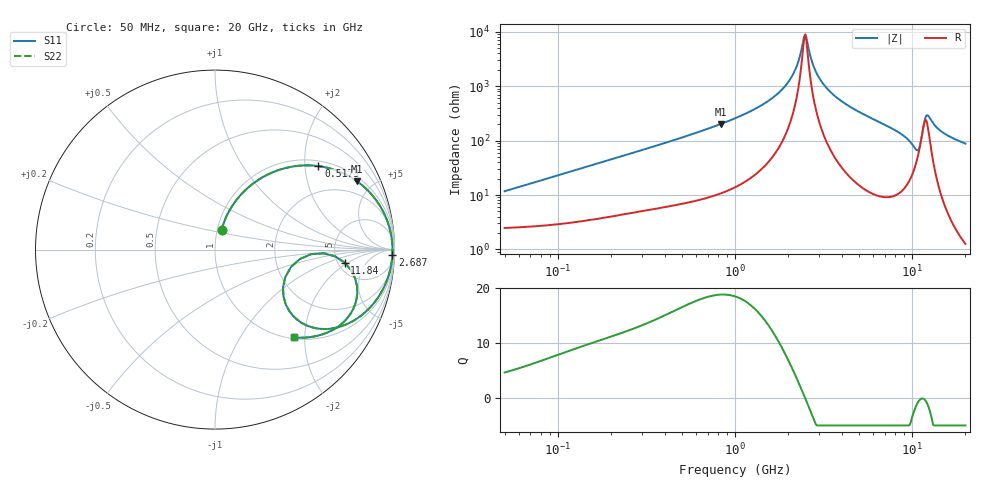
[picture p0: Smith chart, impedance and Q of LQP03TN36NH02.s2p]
!Murata Part Number: LQP03TN36NH02
!These Parameters are Measured in Series Mode Connection
!  o--[Z]--o
!Port1  Port2
!  o-------o
!Freq. Start=50[MHz] Stop=20[GHz], 401[Steps]
# Hz S RI R 50
!Freq.(Hz) S11(Real) S11(Imag) S21(Real) S21(Imag) S12(Real) S12(Imag) S22(Real) S22(Imag)
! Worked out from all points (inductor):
!   401 points, 50 MHz to 20 GHz, reference 50 ohm
!   read as one part in series: L = 36.4 nH near 51.52 MHz
!   highest Q = 18.8 at 835.5 MHz (marker M1), where L = 38.6 nH
!   self-resonance near 2.456 GHz
!   S11 on the Smith chart (normalised r, x): 50 MHz: 1.05, +0.23; 517.3 MHz: 1.14, +2.35; 2.687 GHz: 24, -60; 11.84 GHz: 5.75, -1.77; 20 GHz: 1.03, -1.76
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5e7  0.0363 0.1079  0.9637 -0.1079  0.9637 -0.1079  0.0363 0.1079
1.364002e8  0.1116 0.2661  0.8884 -0.2661  0.8884 -0.2661  0.1116 0.2661
3.721004e8  0.4169 0.4599  0.5831 -0.4599  0.5831 -0.4599  0.4169 0.4599
5.173368e8  0.5761 0.4652  0.4239 -0.4652  0.4239 -0.4652  0.5761 0.4652
8.354841e8  0.7926 0.3798  0.2074 -0.3798  0.2074 -0.3798  0.7926 0.3798
1e9  0.8552 0.3259  0.1448 -0.3259  0.1448 -0.3259  0.8552 0.3259
1.454215e9  0.9447 0.1964  0.0553 -0.1964  0.0553 -0.1964  0.9447 0.1964
1.875929e9  0.9767 0.1038  0.0233 -0.1038  0.0233 -0.1038  0.9767 0.1038
2.179053e9  0.9861 0.0489  0.0139 -0.0489  0.0139 -0.0489  0.9861 0.0489
2.493527e9  0.9889 -0.000672  0.0111 0.000672  0.0111 0.000672  0.9889 -0.000672
2.687447e9  0.9883 -0.0284  0.0117 0.0284  0.0117 0.0284  0.9883 -0.0284
2.728004e9  0.9879 -0.0339  0.0121 0.0339  0.0121 0.0339  0.9879 -0.0339
3.075291e9  0.9829 -0.0785  0.0171 0.0785  0.0171 0.0785  0.9829 -0.0785
3.736399e9  0.9649 -0.1522  0.0351 0.1522  0.0351 0.1522  0.9649 -0.1522
7.442007e9  0.7469 -0.4096  0.2531 0.4096  0.2531 0.4096  0.7469 -0.4096
9.316812e9  0.5436 -0.4339  0.4564 0.4339  0.4564 0.4339  0.5436 -0.4339
1.050288e10  0.3815 -0.261  0.6185 0.261  0.6185 0.261  0.3815 -0.261
1.131968e10  0.537 -0.0251  0.463 0.0251  0.463 0.0251  0.537 -0.0251
1.183995e10  0.7226 -0.0726  0.2774 0.0726  0.2774 0.0726  0.7226 -0.0726
1.257102e10  0.7928 -0.241  0.2072 0.241  0.2072 0.241  0.7928 -0.241
1.417136e10  0.703 -0.4157  0.297 0.4157  0.297 0.4157  0.703 -0.4157
2e10  0.4381 -0.489  0.5619 0.489  0.5619 0.489  0.4381 -0.489
